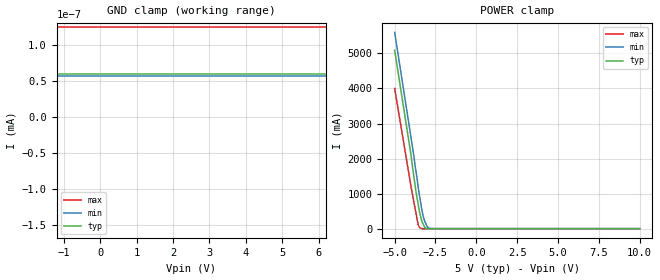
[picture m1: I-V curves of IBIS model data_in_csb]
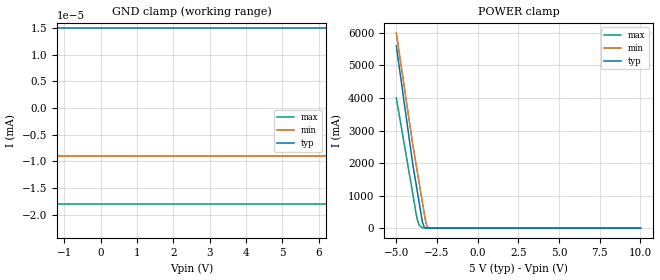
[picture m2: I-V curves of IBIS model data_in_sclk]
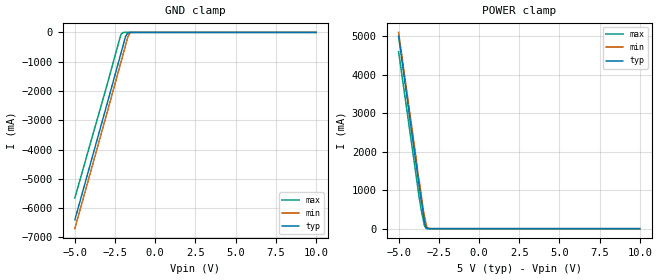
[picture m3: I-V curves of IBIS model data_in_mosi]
[IBIS Ver]   4.0
[File name]   fs23_spi.ibs
[File Rev]   1.1
[Date]   SEPTEMBER 2024
[Source]   NXP semiconductors
[Notes]   IBIS model for the fs23 includes the model of SPI pins
|   (SCLK. CSB. MOSI and MISO).
|   MISO pin model is not representative of the FS24 MISO pin
[Disclaimer]   This information is for modeling purposes only
|   and is not guaranteed.The simulation model is not able to
|   reproduce identically the quality structure
|   and behavior of the final product.
[Copyright]   Copyright 2021 NXP Semiconductors: All Rights Reserved. This
|   simulation model or derivative thereof is the proprietary
|   information of NXP Semiconductors. is confidential in nature
|   and may not be reproduced in any way
|   (physically or electronically)
|   without the express permission from NXP Semiconductors.
[Component]   fs23
[Manufacturer]   NXP semiconductors
[Package]
|   typ   min   max
R_pkg   0.083216   0.072192   0.098491
L_pkg   1.928e-9   1.494e-9   2.406e-9
C_pkg   2.869e-13   2.631e-13   3.056e-13
[Pin]   Signal_name   model_name   R_pin   L_pin   C_pin
28   CSB   data_in_csb   0.072192   1.494e-9   2.631e-13
27   SCK   data_in_sclk   0.075468   1.744e-9   2.79e-13
26   MOSI   data_in_mosi   0.086713   2.067e-9   2.997e-13
25   MISO   data_out_miso   0.098491   2.406e-9   3.056e-13
| end pin list
| Models and submodels in the file (4): data_in_csb (Input), data_in_sclk (Input), data_in_mosi (Input), data_out_miso (Output)
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|   Model data_in_csb
[Model]   data_in_csb
Model_type   Input
Polarity   Non-Inverting
|   typ   min   max
C_comp   86.27f   82.63f   97.24f
| Where typ is typical value of c_comp (no PVT)
|   min is the minimum value of c_comp under PVT
|   max is the maximum value of c_comp under PVT
Vinh  =   2.505
Vinl  =   2.114
| Hysteresis
|   |   Rising Edge   Falling Edge
|   |   Switching Region   oo   o   Switching Region
|   |   |  o   oo  ooooooooo   |
|   |   V o   o   |
| Vinh  - - - - - - - - - - x   o   |
|   |   o   o  |
|   |   o   o |
|   |   o   oV
| Vinl  - - - - - - -  o - - - - - - - - - - - - - - - - - x
|   |   o   o
|   |   o   o
|   |oooooo-----------------------------------------------------oooooooo
||   typ   min   max
[Temperature Range]   27   -40   175
|   typ   min   max
[Voltage Range]   5V   4.8V   5.2V
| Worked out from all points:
|   POWER clamp passes 1 mA (typ) near -3.01 V on its own axis
[GND Clamp]
|Voltage   I(typ)   I(min)  I(max)
-5V       -6.4A      -6.7A      -5.7A
-1.6V     -200mA     -400mA     -10mA
-1.5V     -100mA     -250mA     125pA
-1.4V     -50mA      -150mA     125pA
-1.3V     60pA       -50mA      125pA
-1.2V     60pA       57pA       125pA
10V       60pA       57pA       125pA
[POWER Clamp]
|Voltage   I(typ)   I(min)  I(max)
-5V       5.09A      5.6A       4A
-4V       2.1A       2.6A       1.2A
-3.8V     1.4A       1.99A      700mA
-3.7V     1.07A      1.64A      450mA
-3.55V    660mA      1.15A      100mA
-3.45V    420mA      850mA      20mA
-3.35V    240mA      570mA      1mA
-3.25V    120mA      350mA      366pA
-3.15V    30mA       200mA      366pA
-3V       250pA      50mA       366pA
-2.7V     250pA      432pA      366pA
10V       250pA      432pA      366pA
|   Model data_in_sclk
[Model]   data_in_sclk
Model_type   Input
Polarity   Non-Inverting
|   typ   min   max
C_comp   85.91f   82.40f   97.09f
| Where typ is typical value of c_comp (no PVT)
|   min is the minimum value of c_comp under PVT
|   max is the maximum value of c_comp under PVT
Vinh  =   2.50
Vinl  =   2.11
| Hysteresis
|   |   Rising Edge   Falling Edge
|   |   Switching Region   oo   o   Switching Region
|   |   |  o   oo  ooooooooo   |
|   |   V o   o   |
| Vinh  - - - - - - - - - - x   o   |
|   |   o   o  |
|   |   o   o |
|   |   o   oV
| Vinl  - - - - - - -  o - - - - - - - - - - - - - - - - - x
|   |   o   o
|   |   o   o
|   |oooooo-----------------------------------------------------oooooooo
|   typ   min   max
[Temperature Range]   27   -40   175
|   typ   min   max
[Voltage Range]   5V   4.8V   5.2V
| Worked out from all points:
|   POWER clamp passes 1 mA (typ) near -3.10 V on its own axis
[GND Clamp]
|Voltage   I(typ)   I(min)  I(max)
-5V       -6.4A      -6.7A      -5.7A
-1.6V     -200mA     -400mA     -10mA
-1.5V     -100mA     -250mA     -18nA
-1.4V     -50mA      -150mA     -18nA
-1.3V     15nA       -50mA      -18nA
-1.2V     15nA       -9nA       -18nA
10V       15nA       -9nA       -18nA
[POWER Clamp]
|Voltage   I(typ)   I(min)  I(max)
-5V       5.6A       6A         4A
-4V       2A         2.6A       1.09A
-3.8V     1.4A       2A         480mA
-3.7V     1.1A       1.7A       250mA
-3.6V     800mA      1.4A       100mA
-3.4V     200mA      800mA      15mA
-3.3V     50mA       500mA      5mA
-3.15V    5mA        100mA      2.2nA
-3.1V     1mA        50mA       2.2nA
-2.8V     1.4nA      1.2nA      2.2nA
10V       1.4nA      1.2nA      2.2nA
|   Model data_in_mosi
[Model]   data_in_mosi
Model_type   Input
Polarity   Non-Inverting
|   typ   min   max
C_comp   86.20f   82.58f   97.17f
| Where typ is typical value of c_comp (no PVT)
|   min is the minimum value of c_comp under PVT
|   max is the maximum value of c_comp under PVT
Vinh  =   2.505
Vinl  =   2.114
| Hysteresis
|   |   Rising Edge   Falling Edge
|   |   Switching Region   oo   o   Switching Region
|   |   |  o   oo  ooooooooo   |
|   |   V o   o   |
| Vinh  - - - - - - - - - - x   o   |
|   |   o   o  |
|   |   o   o |
|   |   o   oV
| Vinl  - - - - - - -  o - - - - - - - - - - - - - - - - - x
|   |   o   o
|   |   o   o
|   |oooooo-----------------------------------------------------oooooooo
||   typ   min   max
[Temperature Range]   27   -40   175
|   typ   min   max
[Voltage Range]   5V   4.8V   5.2V
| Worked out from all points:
|   GND clamp passes 1 mA (typ) near -1.60 V on its own axis
|   POWER clamp passes 1 mA (typ) near -3.21 V on its own axis
[GND Clamp]
|Voltage   I(typ)   I(min)  I(max)
-5V       -6.4A      -6.7A      -5.65A
-3V       -2.45A     -2.75A     -1.8A
-2.15V    -750mA     -1.05A     -100mA
-2V       -450mA     -750mA     -10mA
-1.85V    -150mA     -450mA     125pA
-1.7V     -30mA      -150mA     125pA
-1.55V    -1.6pA     -20mA      125pA
10V       -1.6pA     57pA       125pA
[POWER Clamp]
|Voltage   I(typ)   I(min)  I(max)
-5V       5A         5.1A       4.6A
-3.9V     1.65A      1.8A       1.35A
-3.75V    1.2A       1.3A       900mA
-3.7V     1.05A      1.2A       750mA
-3.6V     750mA      900mA      500mA
-3.55V    650mA      750mA      400mA
-3.45V    350mA      450mA      200mA
-3.4V     200mA      350mA      90mA
-3.35V    100mA      250mA      49mA
-3.25V    8mA        50mA       446pA
-3.15V    335pA      10mA       446pA
10V       335pA      533pA      446pA
